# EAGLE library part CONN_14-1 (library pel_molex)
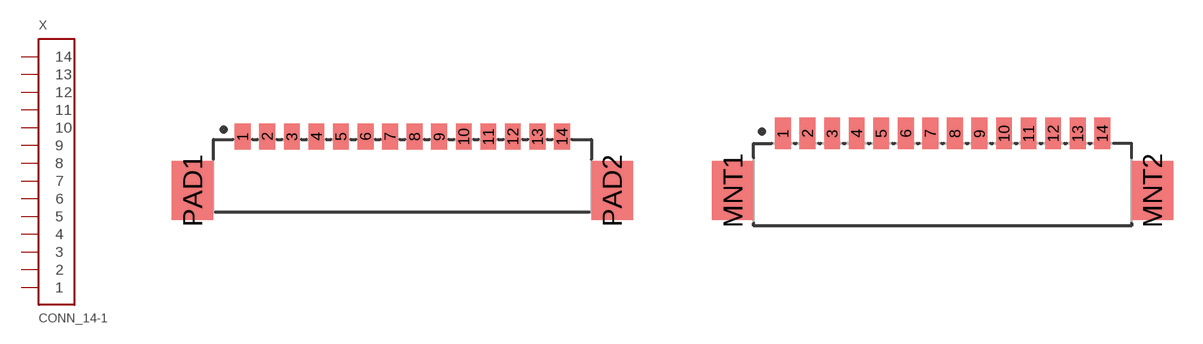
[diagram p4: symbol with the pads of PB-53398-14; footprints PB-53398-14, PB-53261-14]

Designator prefix X

## CONN_14-1-53398  [PB-53398-14]
1  1
2  2
3  3
4  4
5  5
6  6
7  7
8  8
9  9
10  10
11  11
12  12
13  13
14  14

## CONN_14-1-53261  [PB-53261-14]
Pads as for PB-53398-14

## CONN_14-1-53047  [PB-53047-14]
Pads as for PB-53398-14

## Footprint PB-53398-14 (pad centres in mm)
smd 0.8 x 1.3: 1 -8.125,1.25; 2 -6.875,1.25; 3 -5.625,1.25; 4 -4.375,1.25; 5 -3.125,1.25; 6 -1.875,1.25; 7 -0.625,1.25; 8 0.625,1.25; 9 1.875,1.25; 10 3.125,1.25; 11 4.375,1.25; 12 5.625,1.25; 13 6.875,1.25; 14 8.125,1.25
smd 2.1 x 3: PAD1 -10.675,-1.5; PAD2 10.675,-1.5

## Footprint PB-53261-14 (pad centres in mm)
smd 0.8 x 1.6: 1 -8.125,1.1; 2 -6.875,1.1; 3 -5.625,1.1; 4 -4.375,1.1; 5 -3.125,1.1; 6 -1.875,1.1; 7 -0.625,1.1; 8 0.625,1.1; 9 1.875,1.1; 10 3.125,1.1; 11 4.375,1.1; 12 5.625,1.1; 13 6.875,1.1; 14 8.125,1.1
smd 2.1 x 3: MNT1 -10.675,-1.8; MNT2 10.675,-1.8

## Footprint PB-53047-14 (pad centres in mm)
drill 0.5: 1 -8.125,0; 2 -6.875,0; 3 -5.625,0; 4 -4.375,0; 5 -3.125,0; 6 -1.875,0; 7 -0.625,0; 8 0.625,0; 9 1.875,0; 10 3.125,0; 11 4.375,0; 12 5.625,0; 13 6.875,0; 14 8.125,0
